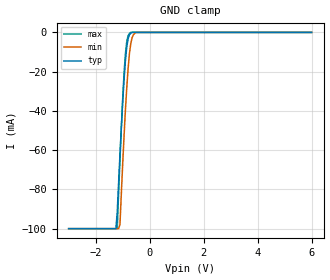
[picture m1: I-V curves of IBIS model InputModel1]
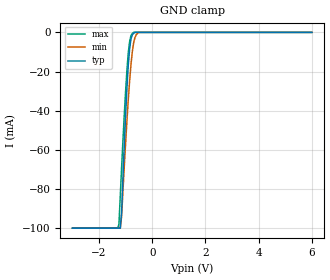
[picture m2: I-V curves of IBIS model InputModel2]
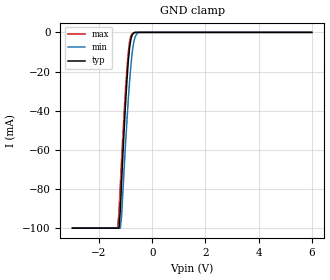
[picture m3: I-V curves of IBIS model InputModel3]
[IBIS Ver]   2.1
[File name]   e_008bel.ibs   | e_= TSOP, f008be= abbr chip name,
|   | l = 2.7 to 3.3V Vcc
[File Rev]   2.00
[Date]   2-April-1996
[Source]   File generated from lab measurements at Intel Corporation
[Notes]   Rev 2.00 All data was replaced by actual measurements
   performed in a lab.
[Disclaimer] INTEL DEVELOPER'S SOFTWARE LICENSE AGREEMENT
| BY USING THIS SOFTWARE, YOU ARE AGREEING TO BE BOUND
| BY THE TERMS OF THIS AGREEMENT.  DO NOT USE THE SOFTWARE
| UNTIL YOU HAVE CAREFULLY READ AND AGREED TO THE FOLLOWING
| TERMS AND CONDITIONS.  IF YOU DO NOT AGREE TO THE TERMS
| OF THIS AGREEMENT, PROMPTLY RETURN THE SOFTWARE PACKAGE
| AND ANY ACCOMPANYING ITEMS.
| IF YOU USE THIS SOFTWARE, YOU WILL BE BOUND BY THE TERMS
| OF THIS AGREEMENT
| LICENSE: Intel Corporation ("Intel") grants you the non-exclusive right
| to use the enclosed software program ("Software").  You will not use,
| copy, modify, rent, sell or transfer the Software or any portion
| thereof, except as provided in this Agreement.
| System OEM Developers may:
| 1.   Copy the Software for support, backup or archival purposes;
| 2.   Install, use, or distribute Intel owned Software in object code
|   only;
| 3.   Modify and/or use Software source code that Intel directly makes
|   available to you as an OEM Developer;
| 4.   Install, use, modify, distribute, and/or make or have made
|   derivatives ("Derivatives") of Intel owned Software under the
|   terms and conditions in this Agreement, ONLY if you are a System
|   OEM Developer and NOT an end-user.
| RESTRICTIONS:
| YOU WILL NOT:
| 1.   Copy the Software, in whole or in part, except as provided for
|   in this Agreement;
| 2.   Decompile or reverse engineer any Software provided in object
|   code format;
| 3.   Distribute any Software or Derivative code to any end-users,
|   unless approved by Intel in a prior writing.
| TRANSFER: You may transfer the Software to another OEM
| Developer if the receiving party agrees to the terms of this
| Agreement at the sole risk of any receiving party.
| OWNERSHIP AND COPYRIGHT OF SOFTWARE:
| Title to the Software and all copies thereof remain with Intel
| or its vendors.  The Software is copyrighted and is protected by
| United States and international copyright laws.  You will not
| remove the copyright notice from the Software.  You agree to
| prevent any unauthorized copying of the Software.
| DERIVATIVE WORK: OEM Developers that make or have made
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[Copyright]   Copyright 1996, Intel Corporation, All Rights Reserved
[Component]   E28F008BE   | 40-lead TSOP package, 28F008BE
[Manufacturer]  Intel   | Boot Block (tm)
|   | operating in 2.7-3.3V Vcc range
[Package]
|Variable   typ   min   max
|The following values apply for the leadframe.
R_pkg   135m   126m   144m
L_pkg   3.95nH   3.62nH   4.28nH
C_pkg   0.39pF   0.38pF   0.40pF
|*****************************Pin Definitions**********************************
[Pin]   signal_name   model_name   R_pin   L_pin   C_pin
 1   A16   InputModel2
 2   A15   InputModel3
 3   A14   InputModel3
 4   A13   InputModel3
 5   A12   InputModel3
 6   A11   InputModel3
 7   A09   InputModel3
 8   A08   InputModel3
 9   WE#   InputModel1
10   RP#   InputModel1
11   VPP   POWER
12   WP#   InputModel1
13   A18   InputModel3
14   A07   InputModel3
15   A06   InputModel3
16   A05   InputModel3
17   A04   InputModel3
18   A03   InputModel3
19   A02   InputModel3
20   A01   InputModel3
21   A00   InputModel2
22   CE#   InputModel1
23   GND   GND
24   OE#   InputModel1
25   DQ0   InputOutput
26   DQ1   InputOutput
27   DQ2   InputOutput
28   DQ3   InputOutput
29   NC   InputModel4
30   VCC   POWER
31   VCC   POWER
32   DQ4   InputOutput
33   DQ5   InputOutput
34   DQ6   InputOutput
35   DQ7   InputOutput
36   A10   InputModel3
37   A19   InputModel3
38   NC   InputModel4
39   GND   GND
40   A17   InputModel3
|***********************Input Model 4******************************
[Model]   InputModel4
Model_type   Input
|   Model for NC pins (Numbers 29, & 38).
Vinl = 0.8V
Vinh = 2.0V
|Variable   Typ   Min   Max
C_comp   5.61p   NA   7.6p
[Voltage Range]   3.0V   2.7V   3.3V
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| Models and submodels in the file (5): InputModel1 (Input), InputModel2 (Input), InputModel3 (Input), InputModel4 (Input), InputOutput (I/O)
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|*********************Input Model 1************************************
[Model]   InputModel1
Model_type   Input
|   Model for WE#, WP#, RP#, OE# & CE#.
Vinl = 0.8V
Vinh = 2.0V
|Variable   Typ   Min   Max
C_comp   5.61p   NA   7.6p
[Voltage Range]   3.0V   2.7V   3.3V
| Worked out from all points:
|   GND clamp passes 1 mA (typ) near -0.74 V on its own axis
[GND_clamp]
|Voltage  I(typ)   I(min)   I(max)
-3V       -100mA     -100mA     -100mA
-1.25V    -100mA     -100mA     -100mA
-1.2V     -91.38mA   -100mA     -99.69mA
-1.1V     -62.33mA   -97.89mA   -64.9mA
-1V       -35.99mA   -67.36mA   -34.11mA
-900mV    -14.83mA   -40.08mA   -11.26mA
-850mV    -7.774mA   -28.73mA   -4.823mA
-800mV    -3.283mA   -18.71mA   -1.668mA
-700mV    -471.4uA   -5.736mA   0A
-600mV    0A         -1.158mA   0A
-500mV    0A         0A         0A
6V        0A         0A         0A
[Power_clamp]
| Input buffer circuits of this product do not intrinsically
| require a [Power_clamp] definition.  This zero current
| [Power_clamp] table is provided for the compatibility with
| some IBIS parsers.
|Voltage  I(typ)   I(min)   I(max)
-3V       0A         0A         0A
0V        0A         0A         0A
3V        0A         0A         0A
6V        0A         0A         0A
|*********************Input Model 2******************************
[Model]   InputModel2
Model_type   Input
|   Model for A[0] & A[16] pins.
Vinl = 0.8V
Vinh = 2.0V
|Variable   Typ   Min   Max
C_comp   5.61p   NA   7.6p
[Voltage Range]   3.0V   2.7V   3.3V
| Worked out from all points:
|   GND clamp passes 1 mA (typ) near -0.73 V on its own axis
[GND_clamp]
|Voltage  I(typ)   I(min)   I(max)
-3V       -100mA     -100mA     -100mA
-1.3V     -100mA     -100mA     -100mA
-1.25V    -100mA     -100mA     -97.92mA
-1.2V     -100mA     -100mA     -83.24mA
-1.15V    -91.8mA    -93.8mA    -68.92mA
-1V       -42.09mA   -56.51mA   -29.98mA
-900mV    -16.78mA   -34.42mA   -10.53mA
-850mV    -8.519mA   -25.07mA   -4.731mA
-800mV    -3.472mA   -16.7mA    -1.714mA
-700mV    -480.5uA   -5.462mA   0A
-500mV    0A         0A         0A
6V        0A         0A         0A
[Power_clamp]
| Input buffer circuits of this product do not intrinsically
| require a [Power_clamp] definition.  This zero current
| [Power_clamp] table is provided for the compatibility with
| some IBIS parsers.
|Voltage  I(typ)   I(min)   I(max)
-3V       0A         0A         0A
0V        0A         0A         0A
3V        0A         0A         0A
6V        0A         0A         0A
|***********************Input Model 3******************************
[Model]   InputModel3
Model_type   Input
|   Model for A[15:1] & A[19:17].
Vinl = 0.8V
Vinh = 2.0V
|Variable   Typ   Min   Max
C_comp   5.61p   NA   7.6p
[Voltage Range]   3.0V   2.7V   3.3V
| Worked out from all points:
|   GND clamp passes 1 mA (typ) near -0.74 V on its own axis
[GND_clamp]
|Voltage  I(typ)   I(min)   I(max)
-3V       -100mA     -100mA     -100mA
-1.3V     -100mA     -100mA     -100mA
-1.25V    -100mA     -100mA     -91.69mA
-1.2V     -90.85mA   -100mA     -78.06mA
-1.15V    -76.19mA   -93.92mA   -64.74mA
-1.05V    -48.54mA   -68.57mA   -39.73mA
-950mV    -24.46mA   -45.15mA   -18.47mA
-850mV    -7.709mA   -25.05mA   -4.698mA
-750mV    -1.198mA   -10.09mA   -626uA
-650mV    0A         -2.645mA   0A
-500mV    0A         0A         0A
6V        0A         0A         0A
[Power_clamp]
| Input buffer circuits of this product do not intrinsically
| require a [Power_clamp] definition.  This zero current
| [Power_clamp] table is provided for the compatibility with
| some IBIS parsers.
|Voltage  I(typ)   I(min)   I(max)
-3V       0A         0A         0A
0V        0A         0A         0A
3V        0A         0A         0A
6V        0A         0A         0A
